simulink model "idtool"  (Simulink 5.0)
settings: Solver=ode45  SolverMode=SingleTasking  StartTime=0.0  StopTime=10  MaxStep=10  RelTol=1e-3  AbsTol=1e-3

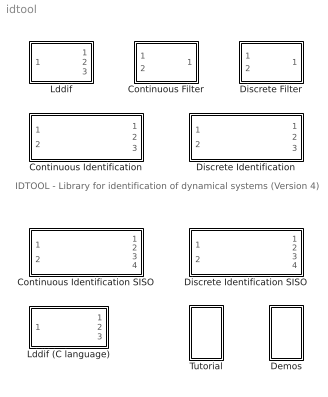
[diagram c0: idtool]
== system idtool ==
  note: IDTOOL - Library for identification of dynamical systems (Version 4)
  Continuous Filter : Subsystem  mask(C-Filter){par=[1,1], cit=[0], men=[1], tc=[1]}
      mask prompts: par "No. of inputs and outputs -  [in,out]:"; cit "Numerator degree -  [dn]:"; men "Denominator degree -  [dd]:"; tc "Time constant of the filter - [Tc]:"
      mask help: C-filter: Continuous filters Authors: Lubos Cirka and Miroslav Fikar 1998 - 2006
      mask init:
      | % State-space realisation of continuous-time MIMO filters
      | %
      | % Input:
      | %    y1(t), ..., yn(t), u1(t), ..., um(t)
      | % Output:
      | %    y(t), y'(t), y''(t) ..., u(t), u'(t), ...
      | 
      | % Calculation of the denominator with multiple time constant tc
      | 
      | in=par(1); out=par(2);
      | den=1;
      | for i=1:men,
      |    den=conv([tc 1],den);
      | end;
      | a=fliplr(den(2:men+1)/den(1));
      | 
      | % State-space realisation of the output filter
      | 
      | A0=zeros(out*(men-1),out);
      | A1=eye(out*(men-1));
      | for i=1:men
      |    A2(1:out,out*(i-1)+1:i*out)=-a(i)*eye(out);
      | end
      | Ay=[A0 A1;A2];
      | B0=zeros(out*(men-1),out);
      | B1=eye(out,out);
      | By=[B0;B1];
      | 
      | C0=-eye(out*(men-1)+out);C0(1:out,1:out)=eye(out);
      | for i=1:men
      |    C1(1:out,out*(i-1)+1:i*out)=a(i)*eye(out);
      | end
      | Cy=[C0;C1]/den(1);
      | Dy=-[zeros(out,out);By]/den(1);
      | 
      | % State-space realisation of the input filter
      | 
      | a0=zeros(in*(men-1),in);
      | a1=eye(in*(men-1));
      | for i=1:men
      |    a2(1:in,in*(i-1)+1:i*in)=-a(i)*eye(in);
      | end
      | Au=[a0 a1;a2];
      | b0=zeros(in*(men-1),in);
      | b1=eye(in,in);
      | Bu=[b0;b1];
      | if cit==men
      |    c0=eye(in*(cit-1)+in);
      |    for i=1:cit
      |       c1(1:in,in*(i-1)+1:i*in)=-a(i)*eye(in);
      |    end
      |    Cu=[c0;c1]/den(1);
      |    Du=[zeros(in*(cit-1)+in,in);eye(in)]/den(1);
      | else
      |    c0=eye(in*(cit+1));
      |    c1=zeros(in*(cit+1),(men-cit-1)*in);
      |    Cu=[c0 c1]/den(1);
      |    Du=zeros(in*(cit+1),in);
      | end
  Continuous Identification : Subsystem  mask(Continuous Identification){par3=[2,2], par1=[0,1], tc=[1], par2=[0.985,0.01], poc=[0 0 0 0 0 0 0 0], kov=[10e6], ts=[1]}
      mask prompts: par3 "Number of inputs and outputs -  [in,out]:"; par1 "Degrees of numerator and denominator -  [dn, dd]:"; tc "Time constant of the filter - [Tc]:"; par2 "Exponential forgetting and Bittanti's correction - [L, d]:"; poc "Initial parameter estimates - [theta(1) ... theta(n)]:"; kov "Covariance matrix (see help, standard - [10e6]):"; ts "Sampling time - [ts]:"
      mask help: Continuous identification Authors: Lubos Cirka and Miroslav Fikar 1998 - 2006
      mask init:
      | % State-space realisation of continuous-time filters
      | %
      | % Input:
      | %    y_1(t), ..., y_in(t), u_1(t), ..., u_out(t)
      | % Output:
      | %    y_1(t), ..., y_in(t), -y_1'(t), ..., -y_in'(t), -y_1''(t), ..., -y_in''(t), ..., 
      | %    u_1(t), ..., u_out(t), u_1'(t), ..., u_out'(t), u_1''(t), ..., u_out''(t), ...
      | 
      | % Parameters definition
      | cit = par1(1); % numerator degree 
      | men = par1(2); % denumerator degree
      | L = par2(1); % exponential forgetting
      | d = par2(2); % Bittanti's correction
      | n = (cit+1)*par3(1)+men*par3(2); % number of data
      | m = par3(2); % 
      | in = par3(1); % number of inputs
      | out = par3(2); % number of outputs
      | 
      | % Calculation of the denominator with multiple time constant tc
      | den = 1;
      | for i = 1:men,
      |    den = conv([tc 1],den);
      | end;
      | a = fliplr(den(2:men+1)/den(1));
      | 
      | % State-space realisation of the output filter ([Ay, By, Cy, Dy])
      | A0 = zeros(out*(men-1),out);
      | A1 = eye(out*(men-1));
      | for i = 1:men
      |    A2(1:out,out*(i-1)+1:i*out) = -a(i)*eye(out);
      | end
      | Ay = [A0 A1;A2];
      | B0 = zeros(out*(men-1),out);
      | B1 = eye(out,out);
      | By = [B0;B1];
      | 
      | C0 = -eye(out*(men-1)+out);
      | C0(1:out,1:out) = eye(out);
      | for i = 1:men
      |    C1(1:out,out*(i-1)+1:i*out) = a(i)*eye(out);
      | end
      | Cy = [C0;C1]/den(1);
      | Dy = -[zeros(out,out);By]/den(1);
      | 
      | % State-space realisation of the input filter ([Au, Bu, Cu, Du])
      | a0 = zeros(in*(men-1),in);
      | a1 = eye(in*(men-1));
      | for i = 1:men
      |    a2(1:in,in*(i-1)+1:i*in) = -a(i)*eye(in);
      | end
      | Au = [a0 a1;a2];
      | b0 = zeros(in*(men-1),in);
      | b1 = eye(in,in);
      | Bu = [b0;b1];
      | if cit==men
      |    c0 = eye(in*(cit-1)+in);
      |    for i = 1:cit
      |       c1(1:in,in*(i-1)+1:i*in) = -a(i)*eye(in);
      |    end
      |    Cu = [c0;c1]/den(1);
      |    Du = [zeros(in*(cit-1)+in,in);eye(in)]/den(1);
      | else
      |    c0 = eye(in*(cit+1));
      |    c1 = zeros(in*(cit+1),(men-cit-1)*in);
      |    Cu = [c0 c1]/den(1);
      |    Du = zeros(in*(cit+1),in);
      | end
  Continuous Identification SISO : Subsystem  mask(Continuous Identification){par1=[1,2], tc=[0.5], par2=[0.985,0.01], poc=[0 0 0 0], kov=[10e6], ts=[1]}
      mask prompts: par1 "Degrees of numerator and denominator -  [dn, dd]:"; tc "Time constant of the filter - [Tc]:"; par2 "Exponential forgetting and Bittanti's correction - [L, d]:"; poc "Initial parameter estimates - [theta(1) ... theta(n)]:"; kov "Covariance matrix (see help, standard - [10e6]):"; ts "Sampling time - [ts]:"
      mask help: Continuous identification Authors: Lubos Cirka and Miroslav Fikar 1998 - 2006
      mask init:
      | % State-space realisation of continuous-time MIMO filters
      | %
      | % Input:
      | %    y1(t), ..., yn(t), u1(t), ..., um(t)
      | % Output:
      | %    y(t), y'(t), y''(t) ..., u(t), u'(t), ...
      | 
      | % Calculation of the denominator with multiple time constant tc
      | 
      | cit=par1(1);men=par1(2);L=par2(1);d=par2(2); n=cit+men+1;m=1;in=1;out=1;
      | den=1;
      | for i=1:men,
      |    den=conv([tc 1],den);
      | end;
      | a=fliplr(den(2:men+1)/den(1));
      | 
      | % State-space realisation of the output filter
      | 
      | A0=zeros(out*(men-1),out);
      | A1=eye(out*(men-1));
      | for i=1:men
      |    A2(1:out,out*(i-1)+1:i*out)=-a(i)*eye(out);
      | end
      | Ay=[A0 A1;A2];
      | B0=zeros(out*(men-1),out);
      | B1=eye(out,out);
      | By=[B0;B1];
      | 
      | C0=-eye(out*(men-1)+out);C0(1:out,1:out)=eye(out);
      | for i=1:men
      |    C1(1:out,out*(i-1)+1:i*out)=a(i)*eye(out);
      | end
      | Cy=[C0;C1]/den(1);
      | Dy=-[zeros(out,out);By]/den(1);
      | 
      | % State-space realisation of the input filter
      | 
      | a0=zeros(in*(men-1),in);
      | a1=eye(in*(men-1));
      | for i=1:men
      |    a2(1:in,in*(i-1)+1:i*in)=-a(i)*eye(in);
      | end
      | Au=[a0 a1;a2];
      | b0=zeros(in*(men-1),in);
      | b1=eye(in,in);
      | Bu=[b0;b1];
      | if cit==men
      |    c0=eye(in*(cit-1)+in);
      |    for i=1:cit
      |       c1(1:in,in*(i-1)+1:i*in)=-a(i)*eye(in);
      |    end
      |    Cu=[c0;c1]/den(1);
      |    Du=[zeros(in*(cit-1)+in,in);eye(in)]/den(1);
      | else
      |    c0=eye(in*(cit+1));
      |    c1=zeros(in*(cit+1),(men-cit-1)*in);
      |    Cu=[c0 c1]/den(1);
      |    Du=zeros(in*(cit+1),in);
      | end
  Demos : Subsystem
  Discrete Filter : Subsystem  mask(D-Filter){par=[1,1], cit=[1], men=[1], ts=[1], Ds=[0]}
      mask prompts: par "No. of inputs and outputs -  [in,out]:"; cit "Numerator degree -  [dn]:"; men "Denominator degree -  [dd]:"; ts "Sampling time - [ts]:"; Ds "Discrete time delay - [D]:"
      mask help: D-filter: Discrete filter Authors: Lubos Cirka and Miroslav Fikar 1998 - 2006
      mask init:
      | % State-space realisation of discete-time MIMO filters
      | %
      | % Input:
      | %    y1(k), ..., yn(k), u1(k), ..., um(k)
      | % Output:
      | %    y(k), y(k-1), y(k-2) ..., u(k-1-Ds), ...
      | 
      | % State-space realisation of the output filter
      | 
      | in=par(1); out=par(2);
      | A0=zeros(men*out);
      | A0(out+1:men*out,1:(men-1)*out)=eye((men-1)*out);
      | Ay=A0;
      | 
      | B0=-eye(out);
      | B1=zeros((men-1)*out,out);
      | By=[B0;B1];
      | 
      | C0=zeros(out,men*out);
      | C1=eye(men*out);
      | Cy=[C0;C1];
      | 
      | D1=eye(out);
      | D2=zeros(men*out,out);
      | Dy=[D1;D2];
      | 
      | % State-space realisation of the input filter
      | 
      | a0=zeros(in,(cit+Ds)*in);
      | a1=eye((cit+Ds-1)*in);
      | a2=zeros((cit+Ds-1)*in,in);
      | Au=[a0;[a1 a2]];
      | 
      | b0=eye(in);
      | b1=zeros((cit+Ds-1)*in,in);
      | Bu=[b0;b1];
      | 
      | c0=zeros(cit*in,Ds*in);
      | c1=eye(cit*in);
      | Cu=[c0 c1];
      | 
      | Du=zeros(cit*in,in);
  Discrete Identification : Subsystem  mask(Discrete Identification){par3=[3,2], par1=[2,1], Ds=[0], par2=[0.985,0.01], poc=zeros(1,16), kov=[10e6], ts=[1]}
      mask prompts: par3 "Number of inputs and outputs -  [in,out]:"; par1 "Degrees of numerator and denominator -  [dn, dd]:"; Ds "Discrete time delay - [D]:"; par2 "Exponential forgetting and Bittanti's correction - [L, d]:"; poc "Initial parameter estimates - [theta(1) ... theta(n)]:"; kov "Covariance matrix (see help, standard - [10e6]):"; ts "Sampling time - [ts]:"
      mask help: Discrete identification Authors: Lubos Cirka and Miroslav Fikar 1998 - 2006
      mask init:
      | % State-space realisation of discete-time filters
      | %
      | % Input:
      | %    y_1(k), ..., y_in(k), u_1(k), ..., u_out(k)
      | % Output:
      | %    y_1(k), ..., y_in(k), -y_1(k-1), ..., -y_in(k-1), -y_1(k-2), ..., -y_in(k-2), ..., 
      | %    u_1(k), ..., u_out(k), u_1(k-1), ..., u_out'(k-1), u_1(k-2), ..., u_out(k-2), ...
      | 
      | % Parameters definition
      | cit = par1(1); % numerator degree 
      | men = par1(2); % denumerator degree
      | L = par2(1); % exponential forgetting
      | d = par2(2); % Bittanti's correction
      | n = cit*par3(1)+men*par3(2); % number of data
      | m = par3(2); % 
      | in = par3(1); % number of inputs
      | out = par3(2); % number of outputs
      | 
      | % State-space realisation of the output filter
      | A0=zeros(men*out);
      | A0(out+1:men*out,1:(men-1)*out)=eye((men-1)*out);
      | Ay=A0;
      | 
      | B0=-eye(out);
      | B1=zeros((men-1)*out,out);
      | By=[B0;B1];
      | 
      | C0=zeros(out,men*out);
      | C1=eye(men*out);
      | Cy=[C0;C1];
      | 
      | D1=eye(out);
      | D2=zeros(men*out,out);
      | Dy=[D1;D2];
      | 
      | % State-space realisation of the input filter
      | 
      | a0=zeros(in,(cit+Ds)*in);
      | a1=eye((cit+Ds-1)*in);
      | a2=zeros((cit+Ds-1)*in,in);
      | Au=[a0;[a1 a2]];
      | 
      | b0=eye(in);
      | b1=zeros((cit+Ds-1)*in,in);
      | Bu=[b0;b1];
      | 
      | c0=zeros(cit*in,Ds*in);
      | c1=eye(cit*in);
      | Cu=[c0 c1];
      | 
      | Du=zeros(cit*in,in);
  Discrete Identification SISO : Subsystem  mask(Discrete Identification){par1=[2,2], Ds=[0], par2=[0.985,0.01], poc=[0 0 0 0], kov=[10e6], ts=[1]}
      mask prompts: par1 "Degrees of numerator and denominator -  [dn, dd]:"; Ds "Discrete time delay - [D]:"; par2 "Exponential forgetting and Bittanti's correction - [L, d]:"; poc "Initial parameter estimates - [theta(1) ... theta(n)]:"; kov "Covariance matrix (see help, standard - [10e6]):"; ts "Sampling time - [ts]:"
      mask help: Discrete identification Authors: Lubos Cirka and Miroslav Fikar 1998 - 2006
      mask init:
      | % State-space realisation of discete-time MIMO filters
      | %
      | % Input:
      | %    y1(k), ..., yn(k), u1(k), ..., um(k)
      | % Output:
      | %    y(k), y(k-1), y(k-2) ..., u(k-1-Ds), ...
      | 
      | % State-space realisation of the output filter
      | 
      | cit=par1(1);men=par1(2);L=par2(1);d=par2(2);n=cit+men;m=1;in=1;out=1;
      | A0=zeros(men*out);
      | A0(out+1:men*out,1:(men-1)*out)=eye((men-1)*out);
      | Ay=A0;
      | 
      | B0=-eye(out);
      | B1=zeros((men-1)*out,out);
      | By=[B0;B1];
      | 
      | C0=zeros(out,men*out);
      | C1=eye(men*out);
      | Cy=[C0;C1];
      | 
      | D1=eye(out);
      | D2=zeros(men*out,out);
      | Dy=[D1;D2];
      | 
      | % State-space realisation of the input filter
      | 
      | a0=zeros(in,(cit+Ds)*in);
      | a1=eye((cit+Ds-1)*in);
      | a2=zeros((cit+Ds-1)*in,in);
      | Au=[a0;[a1 a2]];
      | 
      | b0=eye(in);
      | b1=zeros((cit+Ds-1)*in,in);
      | Bu=[b0;b1];
      | 
      | c0=zeros(cit*in,Ds*in);
      | c1=eye(cit*in);
      | Cu=[c0 c1];
      | 
      | Du=zeros(cit*in,in);
  Lddif : Subsystem  mask(LDDIF){par=[4,1], L=[0.985], d=[0.01], poc=[0 0 0 0], kov=[10e6], ts=[1]}
      mask prompts: par "No. of estimated parameters and outputs - [n,m]:"; L "Exponential forgetting - [L]:"; d "Bittanti's correction - [d]:"; poc "Initial parameter estimates - [theta(1) ... theta(n)]:"; kov "Covariance matrix (see help, standard - [10e6]):"; ts "Sampling period - [ts]:"
      mask help: LDDIF: + Bittanti's corrections Authors: Lubos Cirka and Miroslav Fikar 1998 - 2006
      mask init:
      | n=par(1); m=par(2);
  Lddif (C language) : Subsystem  mask(LDDIF){par=[4,1], L=[0.985], d=[0.01], poc=[0 0 0 0], kov=[10e6], ts=[1]}
      mask prompts: par "No. of estimated parameters and outputs - [n,m]:"; L "Exponential forgetting - [L]:"; d "Bittanti's correction - [d]:"; poc "Initial parameter estimates - [theta(1) ... theta(n)]:"; kov "Covariance matrix (see help, standard - [10e6]):"; ts "Sampling period - [ts]:"
      mask help: LDDIF: + Bittanti's corrections Authors: Lubos Cirka and Miroslav Fikar 1998 - 2006
      mask init:
      | n=par(1); m=par(2);
  Tutorial : Subsystem

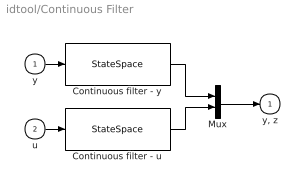
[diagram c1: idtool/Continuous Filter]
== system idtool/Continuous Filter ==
  y : Inport
  u : Inport  Port=2
  Continuous filter - u : StateSpace  A=Au  B=Bu  C=Cu  D=Du
  Continuous filter - y : StateSpace  A=Ay  B=By  C=Cy  D=Dy
  Mux : Mux  Inputs=2
  "y, z" : Outport  InitialOutput=0
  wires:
  Mux/1 -> "y, z"/1
  Continuous filter - u/1 -> Mux/2
  Continuous filter - y/1 -> Mux/1
  u/1 -> Continuous filter - u/1
  y/1 -> Continuous filter - y/1

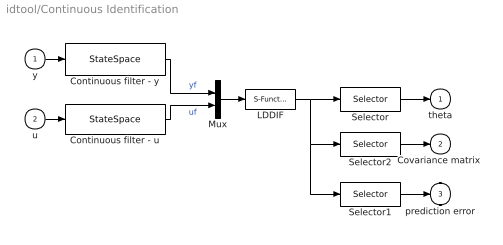
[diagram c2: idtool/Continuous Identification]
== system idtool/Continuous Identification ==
  y : Inport
  u : Inport  Port=2
  Continuous filter - u : StateSpace  A=Au  B=Bu  C=Cu  D=Du
  Continuous filter - y : StateSpace  A=Ay  B=By  C=Cy  D=Dy
  LDDIF : S-Function  FunctionName=lddif_s  Parameters=m, n, L, d, poc, kov, ts
  Mux : Mux  Inputs=2
  Selector : Selector  Elements=[1:1:n*m]  InputPortWidth=n*m+n*n+m
  Selector1 : Selector  Elements=[n*m+n*n+1:1:n*m+n*n+m]  InputPortWidth=n*m+n*n+m
  Selector2 : Selector  Elements=[n*m+1:1:n*m+n*n]  InputPortWidth=n*m+n*n+m
  theta : Outport  InitialOutput=0
  "Covariance matrix " : Outport  Port=2  InitialOutput=0
  prediction error : Outport  Port=3  InitialOutput=0
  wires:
  Selector1/1 -> prediction error/1
  Selector2/1 -> "Covariance matrix "/1
  Selector/1 -> theta/1
  LDDIF/1 -> Selector/1, Selector1/1, Selector2/1
  Mux/1 -> LDDIF/1
  y/1 -> Continuous filter - y/1
  u/1 -> Continuous filter - u/1
  Continuous filter - y/1 -> Mux/1  "yf"
  Continuous filter - u/1 -> Mux/2  "uf"

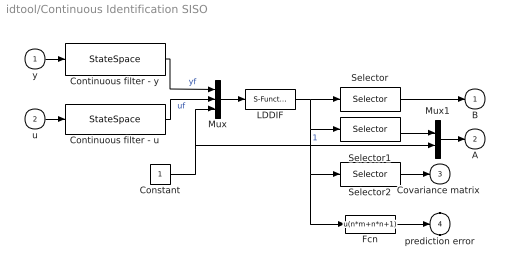
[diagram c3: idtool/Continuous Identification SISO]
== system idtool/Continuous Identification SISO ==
  y : Inport
  u : Inport  Port=2
  Constant : Constant
  Continuous filter - u : StateSpace  A=Au  B=Bu  C=Cu  D=Du
  Continuous filter - y : StateSpace  A=Ay  B=By  C=Cy  D=Dy
  Fcn : Fcn  Expr=u(n*m+n*n+1)
  LDDIF : S-Function  FunctionName=lddif_s  Parameters=m ,n+1 ,L ,d, [poc 0], kov, ts
  Mux : Mux  Inputs=3
  Mux1 : Mux  Inputs=2
  Selector : Selector  Elements=[men+cit+1:-1:men+1]  InputPortWidth=(n+1)*m+(n+1)*(n+1)+m
  Selector1 : Selector  Elements=[men:-1:1]  InputPortWidth=(n+1)*m+(n+1)*(n+1)+m
  Selector2 : Selector  Elements=[(n+1)*m+1:1:(n+1)*m+(n+1)*(n+1)]  InputPortWidth=(n+1)*m+(n+1)*(n+1)+m
  B : Outport  InitialOutput=0
  A : Outport  Port=2  InitialOutput=0
  "Covariance matrix " : Outport  Port=3  InitialOutput=0
  prediction error : Outport  Port=4  InitialOutput=0
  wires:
  Fcn/1 -> prediction error/1
  Selector2/1 -> "Covariance matrix "/1
  Mux1/1 -> A/1
  Selector1/1 -> Mux1/1
  Constant/1 -> Mux1/2, Mux/3  "1"
  Mux/1 -> LDDIF/1
  Selector/1 -> B/1
  y/1 -> Continuous filter - y/1
  u/1 -> Continuous filter - u/1
  Continuous filter - y/1 -> Mux/1  "yf"
  Continuous filter - u/1 -> Mux/2  "uf"
  LDDIF/1 -> Fcn/1, Selector2/1, Selector1/1, Selector/1

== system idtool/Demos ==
  note: Library of demo blocks

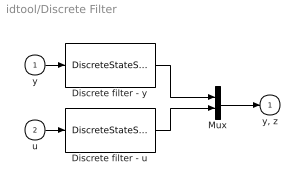
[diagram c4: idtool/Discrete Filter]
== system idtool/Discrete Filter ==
  y : Inport
  u : Inport  Port=2
  Discrete filter - u : DiscreteStateSpace  A=Au  B=Bu  C=Cu  D=Du  SampleTime=ts
  Discrete filter - y : DiscreteStateSpace  A=Ay  B=By  C=Cy  D=Dy  SampleTime=ts
  Mux : Mux  Inputs=2
  "y, z" : Outport  InitialOutput=0
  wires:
  Mux/1 -> "y, z"/1
  Discrete filter - u/1 -> Mux/2
  Discrete filter - y/1 -> Mux/1
  u/1 -> Discrete filter - u/1
  y/1 -> Discrete filter - y/1

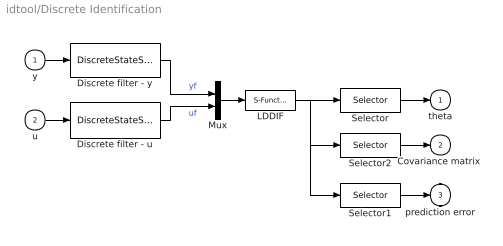
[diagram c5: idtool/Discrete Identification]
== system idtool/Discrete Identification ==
  y : Inport
  u : Inport  Port=2
  Discrete filter - u : DiscreteStateSpace  A=Au  B=Bu  C=Cu  D=Du  SampleTime=ts
  Discrete filter - y : DiscreteStateSpace  A=Ay  B=By  C=Cy  D=Dy  SampleTime=ts
  LDDIF : S-Function  FunctionName=lddif_s  Parameters=m, n, L, d, poc, kov, ts
  Mux : Mux  Inputs=2
  Selector : Selector  Elements=[1:1:n*m]  InputPortWidth=n*m+n*n+m
  Selector1 : Selector  Elements=[n*m+n*n+1:1:n*m+n*n+m]  InputPortWidth=n*m+n*n+m
  Selector2 : Selector  Elements=[n*m+1:1:n*m+n*n]  InputPortWidth=n*m+n*n+m
  theta : Outport  InitialOutput=0
  "Covariance matrix " : Outport  Port=2  InitialOutput=0
  prediction error : Outport  Port=3  InitialOutput=0
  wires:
  LDDIF/1 -> Selector/1, Selector1/1, Selector2/1
  Discrete filter - u/1 -> Mux/2  "uf"
  Discrete filter - y/1 -> Mux/1  "yf"
  u/1 -> Discrete filter - u/1
  y/1 -> Discrete filter - y/1
  Selector/1 -> theta/1
  Mux/1 -> LDDIF/1
  Selector2/1 -> "Covariance matrix "/1
  Selector1/1 -> prediction error/1

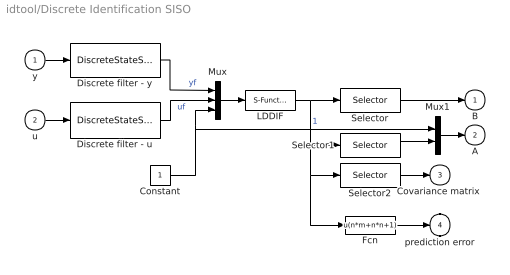
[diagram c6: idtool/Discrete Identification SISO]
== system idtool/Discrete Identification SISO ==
  y : Inport
  u : Inport  Port=2
  Constant : Constant
  Discrete filter - u : DiscreteStateSpace  A=Au  B=Bu  C=Cu  D=Du  SampleTime=ts
  Discrete filter - y : DiscreteStateSpace  A=Ay  B=By  C=Cy  D=Dy  SampleTime=ts
  Fcn : Fcn  Expr=u(n*m+n*n+1)
  LDDIF : S-Function  FunctionName=lddif_s  Parameters=m ,n+1 ,L ,d, [poc 0], kov, ts
  Mux : Mux  Inputs=3
  Mux1 : Mux  Inputs=2
  Selector : Selector  Elements=[men+1:1:men+cit]  InputPortWidth=(n+1)*m+(n+1)*(n+1)+m
  Selector1 : Selector  Elements=[1:1:men]  InputPortWidth=(n+1)*m+(n+1)*(n+1)+m
  Selector2 : Selector  Elements=[(n+1)*m+1:1:(n+1)*m+(n+1)*(n+1)]  InputPortWidth=(n+1)*m+(n+1)*(n+1)+m
  B : Outport  InitialOutput=0
  A : Outport  Port=2  InitialOutput=0
  "Covariance matrix " : Outport  Port=3  InitialOutput=0
  prediction error : Outport  Port=4  InitialOutput=0
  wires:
  LDDIF/1 -> Fcn/1, Selector2/1, Selector1/1, Selector/1
  Discrete filter - u/1 -> Mux/2  "uf"
  Discrete filter - y/1 -> Mux/1  "yf"
  u/1 -> Discrete filter - u/1
  y/1 -> Discrete filter - y/1
  Selector/1 -> B/1
  Mux/1 -> LDDIF/1
  Mux1/1 -> A/1
  Selector2/1 -> "Covariance matrix "/1
  Fcn/1 -> prediction error/1
  Selector1/1 -> Mux1/2
  Constant/1 -> Mux/3, Mux1/1  "1"

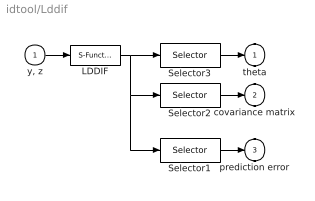
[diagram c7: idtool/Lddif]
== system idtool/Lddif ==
  "y, z" : Inport
  LDDIF : S-Function  FunctionName=lddif_s  Parameters=m, n, L, d, poc, kov, ts
  Selector1 : Selector  Elements=[n*m+n*n+1:1:n*m+n*n+m]  InputPortWidth=n*m+n*n+m
  Selector2 : Selector  Elements=[n*m+1:1:n*m+n*n]  InputPortWidth=n*m+n*n+m
  Selector3 : Selector  Elements=[1:1:n*m]  InputPortWidth=n*m+n*n+m
  theta : Outport  InitialOutput=0
  covariance matrix : Outport  Port=2  InitialOutput=0
  prediction error : Outport  Port=3  InitialOutput=0
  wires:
  "y, z"/1 -> LDDIF/1
  LDDIF/1 -> Selector3/1, Selector2/1, Selector1/1
  Selector2/1 -> covariance matrix/1
  Selector3/1 -> theta/1
  Selector1/1 -> prediction error/1

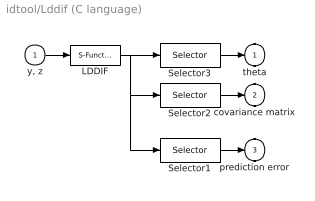
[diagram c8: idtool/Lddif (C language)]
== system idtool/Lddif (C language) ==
  "y, z" : Inport
  LDDIF : S-Function  FunctionName=lddif_s  Parameters=m, n, L, d, poc, kov, ts
  Selector1 : Selector  Elements=[n*m+n*n+1:1:n*m+n*n+m]  InputPortWidth=n*m+n*n+m
  Selector2 : Selector  Elements=[n*m+1:1:n*m+n*n]  InputPortWidth=n*m+n*n+m
  Selector3 : Selector  Elements=[1:1:n*m]  InputPortWidth=n*m+n*n+m
  theta : Outport  InitialOutput=0
  covariance matrix : Outport  Port=2  InitialOutput=0
  prediction error : Outport  Port=3  InitialOutput=0
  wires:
  Selector1/1 -> prediction error/1
  Selector3/1 -> theta/1
  Selector2/1 -> covariance matrix/1
  LDDIF/1 -> Selector1/1, Selector2/1, Selector3/1
  "y, z"/1 -> LDDIF/1

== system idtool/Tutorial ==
  note: Simulations used in tutorial for continuous time identification Simulations used in tutorial for discrete time identification
